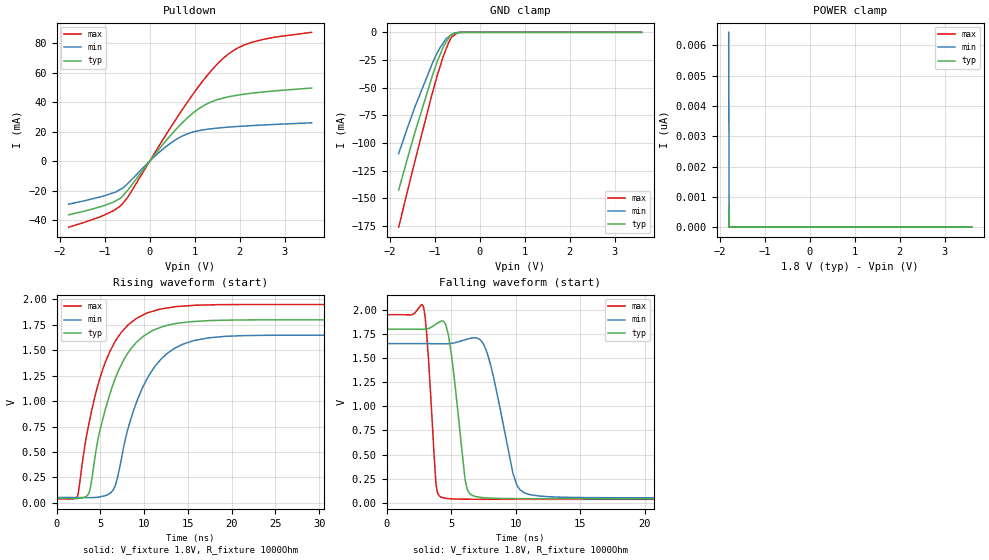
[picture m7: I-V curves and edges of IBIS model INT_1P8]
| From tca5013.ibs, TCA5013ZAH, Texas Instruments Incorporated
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|   Model INT
[Model]   INT_1P8
Model_type   Open_drain
Polarity   Non-Inverting
Vmeas = 0.9
Vref = 1.8
Cref = 15pF
Rref = 1000
|   typ   min   max
C_comp   1.983p   1.522p   2.375p
|C_comp (Low state)   1.922p   1.492p   2.318p
|C_comp (High state)   1.983p   1.522p   2.375p
[Voltage Range]   1.8   1.65   1.95
[Temperature Range]   27   125   -40
[Pullup Reference]   1.8   1.65   1.95
[Pulldown Reference]   0   0   0
[Power Clamp Reference]   1.8   1.65   1.95
[GND Clamp Reference]   0   0   0
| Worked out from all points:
|   slope of the pulldown table from 0 to 0.27 V, typ, clamps not added: 25.7 ohm
|   GND clamp passes 1 mA (typ) near -0.56 V on its own axis
|   falling waveform, V_fixture 1.8V, R_fixture 1000Ohm: 20-80 % time 854ps typ, 1.45ns min, 510ps max; typ from 1.8 V to 0.042 V
|   rising waveform, V_fixture 1.8V, R_fixture 1000Ohm: 20-80 % time 3.68ns typ, 3.88ns min, 3.58ns max; typ from 0.042 V to 1.8 V
[Pulldown]
|   Voltage   I(typ)   I(min)   I(max)
-1.8V     -36.4mA    -29.14mA   -44.79mA
-1.078V   -30.78mA   -24.07mA   -37.54mA
-617.4mV  -24.28mA   -18.55mA   -29.39mA
-487.8mV  -19.75mA   -15.18mA   -24.51mA
198mV     7.764mA    5.673mA    9.909mA
651.6mV   23.8mA     15.9mA     31.65mA
1.181V    37.41mA    21.25mA    54.48mA
1.483V    41.59mA    22.43mA    65.36mA
1.71V     43.47mA    23.06mA    71.84mA
1.98V     45mA       23.66mA    77.24mA
2.304V    46.33mA    24.26mA    81.09mA
3.6V      49.72mA    26.09mA    87.57mA
[GND Clamp]
|   Voltage   I(typ)   I(min)   I(max)
-1.8V     -142.5mA   -109.5mA   -176.2mA
-1.438V   -90.41mA   -67.4mA    -116.3mA
-1.028V   -36.42mA   -25.8mA    -51.43mA
-882mV    -20.53mA   -14.02mA   -31.23mA
-806.4mV  -12.98mA   -9.406mA   -21.45mA
-752.4mV  -9.345mA   -6.108mA   -15.83mA
-693mV    -5.342mA   -4.208mA   -9.637mA
-660.6mV  -3.158mA   -3.171mA   -6.972mA
-617.4mV  -1.653mA   -1.789mA   -4.081mA
-487.8mV  -114.1uA   -350.3uA   -298.5uA
-379.8mV  -6.637uA   -44.44uA   -11.09uA
3.6V      0A         0A         0A
[POWER Clamp]
|   Voltage   I(typ)   I(min)   I(max)
-1.8V     698.2pA    6.43nA     526.8pA
-1.789V   0A         0A         0A
-1.784V   0A         0A         0A
3.6V      0A         0A         0A
[Ramp]
R_load = 1000
|   typ   min   max
dV/dt_r   1.05465/3.6771e-09   0.958608/3.88365e-09   1.14841/3.58333e-09
dV/dt_f   1.05465/8.53976e-10   0.958692/1.45372e-09   1.14841/5.10318e-10
[Falling Waveform]
V_fixture = 1.8V
V_fixture_min = 1.65V
V_fixture_max = 1.95V
R_fixture = 1000Ohm
C_fixture = 0F
|   Time   V(typ)   V(min)   V(max)
0s        1.8V       1.65V      1.95V
2.866ns   1.798V     1.65V      2.03V
3.825ns   1.852V     1.649V     201.9mV
4.29ns    1.884V     1.649V     55.62mV
5.034ns   1.529V     1.653V     41.01mV
6.087ns   236.4mV    1.69V      37.2mV
6.863ns   66.29mV    1.711V     36.52mV
9.792ns   43.52mV    303.2mV    36.21mV
11ns      42.69mV    88.58mV    36.16mV
49.9ns    42.25mV    52.18mV    35.99mV
[Rising Waveform]
V_fixture = 1.8V
V_fixture_min = 1.65V
V_fixture_max = 1.95V
R_fixture = 1000Ohm
C_fixture = 0F
|   Time   V(typ)   V(min)   V(max)
0s        42.25mV    52.17mV    35.99mV
2.407ns   42mV       51.35mV    67.96mV
3.693ns   93.89mV    50.92mV    775.8mV
4.787ns   646.2mV    55.62mV    1.175V
6.425ns   1.156V     119.7mV    1.543V
8.31ns    1.491V     773.9mV    1.759V
10.32ns   1.66V      1.216V     1.866V
13.42ns   1.76V      1.516V     1.926V
17.35ns   1.791V     1.622V     1.946V
49.9ns    1.8V       1.65V      1.95V
